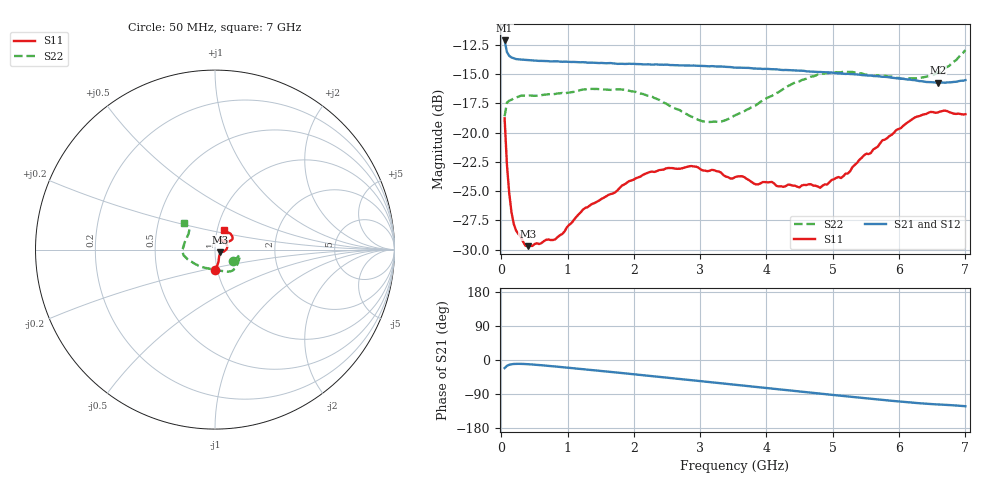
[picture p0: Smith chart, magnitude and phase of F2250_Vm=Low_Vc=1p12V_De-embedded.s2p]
! Integrated Device Technology
! Corporate Headquarters
! 6024 Silver Creek Valley Road
! San Jose, CA 95138  USA
! Phone:  1-408-284-8200
! Toll Free:  1-800-223-1366
! Webpage:  http://www.idt.com/
! Timing and RF Division
! 515 Groton Road, Suite 102
! Westford, MA 01886-6024
! Device:  F2250
! Description: Voltage Variable RF Attenuator
! Frequency:  50.0 -  6000.00 MHz
! Package:  3x3 mm Thin QFN Plastic Package: 16 pin
! Ports:  2 RF, 3 DC
!  Pin  1  = GND
!  Pin  2  = NC
!  Pin  3  = RF1  = Port 1
!  Pin  4  = NC
!  Pin  5  = GND
!  Pin  6  = GND
!  Pin  7  = GND
!  Pin  8  = GND
!  Pin  9  = NC
!  Pin 10  = RF2  = Port 2
!  Pin 11  = NC
!  Pin 12  = GND
!  Pin 13  = GND
!  Pin 14  = VCNTRL
!  Pin 15  = VDD
!  Pin 16  = VMODE
! Vcntrl:  1.120 Volts
! Vmode:  +0.000 Volts
! Vdd:  +3.30  Volts
! Current:  1.191 mA
! Data:  The device was measured on a the F2250 evaluation board which has
!  individual transmission lines to the RF pins.  Data was collected
!  using a calibrated network analyzer.  The evaluation board was
!  de-embedded using a TRL calibration technique.
!  The reference plane is the edge of the package pin.
! Misc:  SN 10
!  Action Tracker AT0258
! Date Measured:  2014-11-26
! Date:  2015-10-15  MJV
! Note:
!  Integrated Device Technology supplies this data as a sample of measured
!  data at the package pin for this product.  Your particular data for this
!  product may vary.
!  Data was taken at 25 degrees C.
!  Integrated Device Technology reserves the right to change this data at anytime.
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# GHz S dB R 50
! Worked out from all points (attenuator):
!   201 points, 50 MHz to 7 GHz, reference 50 ohm
!   highest |S21| = -12.14 dB at 50 MHz (marker M1); lowest = -15.8 dB at 6.583 GHz (marker M2)
!   lowest |S11| = -29.7 dB at 397.5 MHz (marker M3), VSWR 1.07, Z = 52.9 - j1.71 ohm
!   |S11| at or under -10 dB: start of sweep to end of sweep
!   |S22| runs from -19.1 to -13.0 dB; largest |S21 - S12| = 0.00074
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0.05  -18.79 -89.3  -12.14 -21.4  -12.16 -21.4  -18.62 -33.5
0.08475  -22.72 -74.9  -13.13 -15.5  -13.14 -15.5  -17.46 -17.9
0.1195  -25.18 -66.8  -13.45 -12.6  -13.46 -12.7  -17.28 -13.6
0.15425  -26.83 -60.1  -13.59 -11.2  -13.60 -11.2  -17.20 -12.4
0.22375  -28.39 -45.9  -13.73 -10.2  -13.74 -10.2  -17.02 -12.6
0.3975  -29.70 -29.6  -13.81 -11.0  -13.82 -11.0  -16.84 -14.7
0.8145  -29.11 -17.5  -13.92 -17.1  -13.91 -17.1  -16.71 -27.1
1.2315  -26.58 -14.4  -14.00 -24.2  -14.00 -24.2  -16.33 -38.0
1.857  -24.43 -2.1  -14.14 -35.1  -14.14 -35.1  -16.35 -50.6
2.37825  -23.21 10.1  -14.21 -44.4  -14.20 -44.4  -17.20 -62.5
2.86475  -22.86 25.3  -14.29 -53.2  -14.27 -53.2  -18.63 -82.0
3.0385  -23.24 31.5  -14.32 -56.4  -14.31 -56.4  -19.04 -91.7
3.3165  -23.43 41.8  -14.36 -61.5  -14.36 -61.5  -19.06 -109.9
3.525  -23.81 47.9  -14.46 -65.3  -14.44 -65.3  -18.53 -122.7
3.83775  -24.42 59.0  -14.54 -70.9  -14.51 -71.0  -17.68 -139.1
4.7065  -24.53 61.5  -14.81 -86.8  -14.80 -86.8  -15.20 -167.7
4.81075  -24.72 57.5  -14.83 -88.7  -14.83 -88.7  -14.99 -169.7
5.1235  -23.89 47.6  -14.96 -94.3  -14.96 -94.4  -14.85 -176.7
5.85325  -20.30 29.8  -15.29 -107.0  -15.30 -107.1  -15.24 166.3
6.2355  -18.72 32.0  -15.53 -113.1  -15.55 -113.1  -15.38 153.6
6.583  -18.29 41.3  -15.76 -117.3  -15.75 -117.3  -14.85 142.6
7  -18.44 65.4  -15.53 -122.0  -15.54 -122.0  -12.96 139.5
